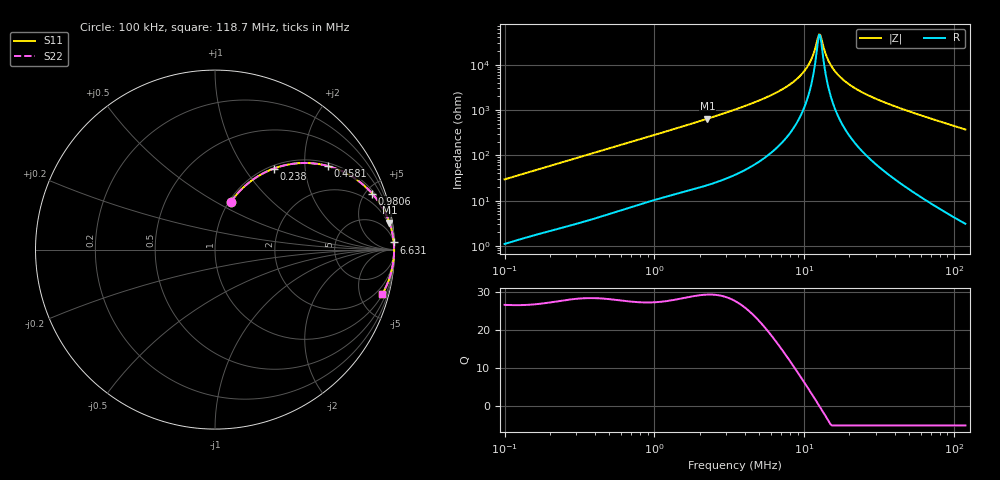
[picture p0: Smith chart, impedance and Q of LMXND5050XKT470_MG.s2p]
! LMXND5050XKT470_MG  S-PARAMETER MODEL  ( General Type )
! Model Generated by TAIYO YUDEN Corporation (https://www.yuden.co.jp/en/)
! Version 1.0
! TAIYO YUDEN Control No. 191023NI43SB-FBB
! Copyright(c) 2019 TAIYO YUDEN CO.,LTD. All Rights Reserved.
! Product Description (link to TY-COMPAS)
! https://ds.yuden.co.jp/TYCOMPAS/or/detail?pn=LMXND5050XKT470MMG&u=M
! Products Name : Inductors
! Characteristics :
!  Inductance : 47 uH , SRF(min) : 9.0 MHz , DC Resistance(max) : 0.4225 Ohm
!  Rated Current : Saturation :950 mA , Temp Rise : 700 mA (40 degC)
!  Case Size : 4.9 x 4.9 / 0.193 x 0.193 [mm/inch] , Thickness : 3 / 0.118 [mm/inch]
!  (Conditions: Temperature = 25 degC , DC Bias Current/Voltage = 0A / 0V)
! External Node Assignments :
!  1  o---GGG---o  2
! GND o---------o GND
! Frequency Range : 0.1MHz  -  118.695536MHz  [ 402 STEP ]
# MHz S RI R 50
! Freq[MHz].  S11 Real  S11 Imag  S21 Real  S21 Imag  S12 Real  S12 Imag  S22 Real  S22 Imag
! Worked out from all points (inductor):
!   401 points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, 100 kHz to 118.7 MHz, reference 50 ohm
!   read as one part in series: L = 46.6 uH near 103.6 kHz
!   highest Q = 29.2 at 2.253 MHz (marker M1), where L = 45.2 uH
!   self-resonance near 12.54 MHz
!   S11 on the Smith chart (normalised r, x): 100 kHz: 1.02, +0.59; 238 kHz: 1.05, +1.38; 458.1 kHz: 1.09, +2.62; 980.6 kHz: 1.20, +5.52; 6.631 MHz: 4, +50; 118.7 MHz: 1.06, -7.43
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0.1  0.0885 0.2658  0.9115 -0.2658  0.9115 -0.2658  0.0885 0.2658
0.155651  0.1802 0.3661  0.8198 -0.3661  0.8198 -0.3661  0.1802 0.3661
0.238023  0.3273 0.4515  0.6727 -0.4515  0.6727 -0.4515  0.3273 0.4515
0.327316  0.4705 0.4817  0.5295 -0.4817  0.5295 -0.4817  0.4705 0.4817
0.458145  0.627 0.4662  0.373 -0.4662  0.373 -0.4662  0.627 0.4662
0.98063  0.8754 0.3124  0.1246 -0.3124  0.1246 -0.3124  0.8754 0.3124
1.07136  0.8924 0.2921  0.1076 -0.2921  0.1076 -0.2921  0.8924 0.2921
2.252948  0.9713 0.1507  0.0287 -0.1507  0.0287 -0.1507  0.9713 0.1507
3.445222  0.9871 0.0963  0.0129 -0.0963  0.0129 -0.0963  0.9871 0.0963
6.631356  0.996 0.0397  0.00401 -0.0397  0.00401 -0.0397  0.996 0.0397
9.281924  0.9975 0.018  0.00255 -0.018  0.00255 -0.018  0.9975 0.018
10.32178  0.9977 0.0117  0.00231 -0.0117  0.00231 -0.0117  0.9977 0.0117
11.27678  0.9978 0.00655  0.00219 -0.00655  0.00219 -0.00655  0.9978 0.00655
12.32013  0.9979 0.00143  0.00213 -0.00143  0.00213 -0.00143  0.9979 0.00143
12.76402  0.9979 -0.000609  0.00211 0.000609  0.00211 0.000609  0.9979 -0.000609
13.94498  0.9979 -0.00572  0.00213 0.00572  0.00213 0.00572  0.9979 -0.00572
14.70538  0.9978 -0.00881  0.00216 0.00881  0.00216 0.00881  0.9978 -0.00881
15.78413  0.9978 -0.013  0.00224 0.013  0.00224 0.013  0.9978 -0.013
17.55242  0.9976 -0.0193  0.00243 0.0193  0.00243 0.0193  0.9976 -0.0193
23.71377  0.9965 -0.0387  0.00354 0.0387  0.00354 0.0387  0.9965 -0.0387
36.91074  0.9925 -0.074  0.00755 0.074  0.00755 0.074  0.9925 -0.074
118.6955  0.9307 -0.2499  0.0693 0.2499  0.0693 0.2499  0.9307 -0.2499
